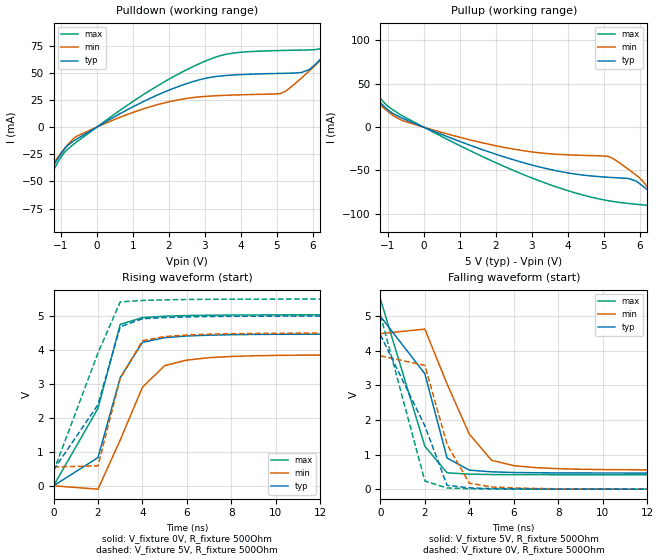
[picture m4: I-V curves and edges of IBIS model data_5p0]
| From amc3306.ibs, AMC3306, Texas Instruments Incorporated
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|   data_5p0 Model
[Model]   data_5p0
Model_type   Output
Polarity   Non-Inverting
Vmeas = 2.5
Vref = 0
Cref = 1pF
Rref = 100000
|   typ   min   max
|   (nom PVT)   (fast PVT)   (slow PVT)
C_comp   1.01pF   1.01pF   1.27pF
| Where Nom  PVT is Nominal Process, 5V, 25C
|   Fast PVT is Strong Process,  5.5V, -40C
|   Slow PVT is Weak Process,   4.5V, 125C
|[Voltage Range]   5   4.5   5.5
[Temperature Range]   25   125   -40
[Pullup Reference]   5   4.5   5.5
[Pulldown Reference]   0   0   0
[Power Clamp Reference]   5   4.5   5.5
[GND Clamp Reference]   0   0   0
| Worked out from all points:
|   slope of the pulldown table from 0 to 0.75 V, typ, clamps not added: 52.6 ohm
|   slope of the pullup table from 0 to 0.75 V, typ, clamps not added: 60.2 ohm
|   falling waveform, V_fixture 5V, R_fixture 500Ohm: 20-80 % time 1.71ns typ, 1.75ns min, 1.43ns max; typ from 5 V to 0.467 V
|   rising waveform, V_fixture 0V, R_fixture 500Ohm: 20-80 % time 1.35ns typ, 1.68ns min, 1.82ns max; typ from 0 V to 4.47 V
|   rising waveform, V_fixture 5V, R_fixture 500Ohm: 20-80 % time 1.8ns typ, 1.2ns min, 1.8ns max; typ from 0.467 V to 5 V
|   falling waveform, V_fixture 0V, R_fixture 500Ohm: 20-80 % time 1.87ns typ, 1.25ns min, 1.26ns max; typ from 4.47 V to 0 V
[Pulldown]
|   Voltage   I(typ)   I(min)   I(max)
-5V       -283.5mA   -269.4mA   -319.1mA
-2.285V   -97.62mA   -97.99mA   -106.9mA
-2.075V   -83.72mA   -84.95mA   -93.21mA
-1.04V    -26.97mA   -25.85mA   -30mA
-605mV    -11.86mA   -9.313mA   -14.74mA
1.48V     26.5mA     18.75mA    33.86mA
3.16V     45.88mA    28.63mA    62.8mA
5.125V    49.5mA     31.26mA    70.59mA
5.89V     52.89mA    51.56mA    71.1mA
6.475V    71.75mA    72.18mA    75.14mA
7.195V    97.47mA    105.3mA    102.7mA
10V       340.3mA    320.9mA    360.5mA
[Pullup]
|   Voltage   I(typ)   I(min)   I(max)
-5V       320.2mA    232.1mA    423.2mA
-3.44V    142.6mA    125.4mA    170.9mA
-2.27V    78.44mA    71.53mA    91.74mA
-1.25V    30.27mA    27.23mA    35.53mA
-620mV    10.82mA    8.11mA     13.75mA
3.205V    -45.83mA   -29.56mA   -61.84mA
5.26V     -58.17mA   -36.44mA   -85.77mA
5.89V     -62.11mA   -55.16mA   -88.92mA
6.46V     -81.05mA   -83.84mA   -93.5mA
7.21V     -107.7mA   -130.2mA   -123.1mA
7.405V    -116.8mA   -142.4mA   -131.3mA
10V       -292.8mA   -306.7mA   -293.7mA
[Ramp]
R_load = 500
|   typ   min   max
dV/dt_r   2.68073/1.34658e-09   2.3138/2.56958e-09   3.02127/1.82299e-09
dV/dt_f   2.71983/1.71419e-09   2.36778/2.70687e-09   3.04931/1.43214e-09
[Falling Waveform]
V_fixture = 5V
V_fixture_min = 4.5V
V_fixture_max = 5.5V
R_fixture = 500Ohm
C_fixture = 0F
|   Time   V(typ)   V(min)   V(max)
0s        5V         4.5V       5.5V
2ns       3.339V     4.631V     1.242V
3ns       900.4mV    3.042V     473.1mV
4ns       550.4mV    1.594V     435.2mV
5ns       501.7mV    836.2mV    423.6mV
6ns       482.5mV    680.4mV    419.8mV
8ns       470.5mV    593mV      418.1mV
15ns      467mV      554.7mV    417.8mV
100ns     467mV      553.7mV    417.8mV
[Rising Waveform]
V_fixture = 0V
V_fixture_min = 0V
V_fixture_max = 0V
R_fixture = 500Ohm
C_fixture = 0F
|   Time   V(typ)   V(min)   V(max)
0s        4.729nV    105.5nV    9.93nV
2ns       830.7mV    -99.21mV   2.28V
3ns       3.187V     1.348V     4.755V
4ns       4.225V     2.903V     4.954V
5ns       4.363V     3.54V      4.996V
6ns       4.413V     3.703V     5.015V
7ns       4.436V     3.774V     5.024V
8ns       4.45V      3.809V     5.029V
10ns      4.462V     3.84V      5.033V
100ns     4.468V     3.856V     5.035V
[Rising Waveform]
V_fixture = 5V
V_fixture_min = 4.5V
V_fixture_max = 5.5V
R_fixture = 500Ohm
C_fixture = 0F
|   Time   V(typ)   V(min)   V(max)
0s        467mV      553.7mV    417.8mV
2ns       2.388V     587.3mV    3.912V
3ns       4.684V     3.159V     5.416V
4ns       4.919V     4.273V     5.459V
5ns       4.955V     4.396V     5.477V
7ns       4.985V     4.466V     5.493V
15ns      5V         4.499V     5.5V
100ns     5V         4.5V       5.5V
[Falling Waveform]
|Gnd
V_fixture = 0V
V_fixture_min = 0V
V_fixture_max = 0V
R_fixture = 500Ohm
C_fixture = 0F
|   Time   V(typ)   V(min)   V(max)
0s        4.468V     3.856V     5.035V
2ns       1.832V     3.582V     237.2mV
3ns       109.1mV    1.296V     34.91mV
4ns       37.99mV    173mV      11.76mV
5ns       16.77mV    62.97mV    4.001mV
7ns       3.693mV    20.17mV    542.8uV
14ns      28.57uV    484.5uV    3.585uV
100ns     3.26uV     121nV      1.895uV
